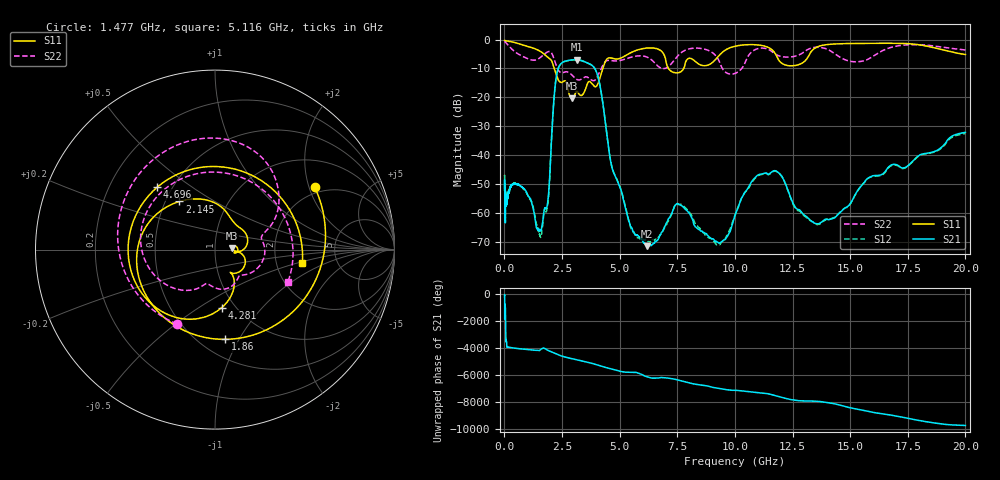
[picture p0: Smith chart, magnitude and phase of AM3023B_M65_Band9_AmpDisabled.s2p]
!Agilent Technologies,E8364B,MY43040894,A.07.50.67
!Agilent E8364B: A.07.50.67
!Date: Tuesday, October 27, 2020 10:50:29
!Correction: S11(Full 2 Port(1,2))
!S21(Full 2 Port(1,2))
!S12(Full 2 Port(1,2))
!S22(Full 2 Port(1,2))
!S2P File: Measurements: S11, S21, S12, S22:Log Frequency Sweep
# Hz S  dB  R 50
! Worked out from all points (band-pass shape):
!   3201 points, 10 MHz to 20 GHz, reference 50 ohm
!   highest |S21| = -6.93 dB at 3.136 GHz (marker M1); lowest = -71.6 dB at 6.201 GHz (marker M2)
!   |S21| within 3 dB of the highest: 2.338 GHz to 3.917 GHz (1.579 GHz wide, 50.5 % of centre)
!   lowest |S11| = -20.4 dB at 2.934 GHz (marker M3), VSWR 1.21, Z = 60.5 + j1.12 ohm
!   |S11| at or under -10 dB: 2.164 GHz to 4.271 GHz (2.107 GHz wide, 65.5 % of centre); 7.121 GHz to 7.779 GHz (658.5 MHz wide, 8.84 % of centre)
!   |S22| runs from -14.2 to -0.6 dB; largest |S21 - S12| = 0.007
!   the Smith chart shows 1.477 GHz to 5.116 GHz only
!   S11 on the Smith chart (normalised r, x): 1.477 GHz: 1.80, +2.18; 1.86 GHz: 0.65, -0.88; 2.145 GHz: 0.59, +0.36; 4.281 GHz: 0.87, -0.63; 4.696 GHz: 0.42, +0.37; 5.116 GHz: 2.82, -0.54
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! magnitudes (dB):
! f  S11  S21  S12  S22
! 10 MHz  -0.3  -52.1  -47.3  -0.6
! 35.55 MHz  -0.3  -61.7  -61.9  -0.8
! 126.1 MHz  -0.5  -54.1  -54.9  -1.6
! 447.2 MHz  -1.0  -49.9  -49.7  -4.1
! 1.477 GHz  -3.7  -65.7  -66.4  -6.6
! 1.59 GHz  -4.2  -66.1  -68.2  -6.0
! 1.86 GHz  -6.0  -57.5  -58.4  -4.3
! 2.145 GHz  -9.5  -21.3  -21.3  -6.5
! 2.364 GHz  -14.3  -9.4  -9.5  -10.9
! 2.934 GHz  -20.4  -7.0  -7.1  -12.3
! 3.136 GHz  -17.9  -6.9  -7.0  -13.8
! 3.902 GHz  -16.2  -9.8  -9.8  -14.2
! 4.281 GHz  -9.7  -22.5  -22.5  -8.8
! 4.696 GHz  -6.5  -45.1  -45.0  -7.3
! 5.116 GHz  -6.1  -53.8  -53.5  -7.0
! 5.639 GHz  -4.0  -67.1  -67.2  -5.8
! 6.201 GHz  -2.9  -71.6  -69.9  -6.1
! 7.588 GHz  -11.4  -57.2  -57.0  -5.1
! 9.375 GHz  -5.0  -70.4  -70.7  -8.6
! 11.44 GHz  -2.7  -46.7  -46.8  -3.4
! 13.91 GHz  -1.8  -62.3  -62.6  -3.0
! 20 GHz  -5.2  -32.1  -32.6  -3.6
